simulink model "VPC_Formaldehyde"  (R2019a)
settings: Solver=VariableStepAuto  StartTime=0.0  StopTime=tend  RelTol=1e-3
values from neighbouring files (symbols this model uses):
  c_MeOH_0 = m_MeOH_sp_0/(m_MeOH_sp_0+m_air_sp_0)    [Mixer_script.m]
  comp_actuator_0 = [z0actuator,comp_w0]    [Compressor_script.m]
  comp_actuator_par = [comp_act_Ga;comp_act_tau;comp_act_zeta]    [Compressor_script.m]
  comp_deltaP = 2.1    [Compressor_script.m]
  comp_p1 = [a0,a1,a2,a3,b0,b1,b2,c0,c1,c2]    [Compressor_script.m]
  comp_p2 = [rho_a, kappa_a, cp_a, R_a, T_amb, d_c]    [Compressor_script.m]
  I_0_compressor = 0.39275    [Compressor_script.m]
  I_0_valve = valve_z0/valve_act_Ga    (= 0.7)    [Valve_script.m]
  Kc_comp = tau_compfotd/(K_compfotd*(tauc_comp+theta_compfotd))    [Compressor_script.m]
  Kc_mtot_MeOH = tau_mtot_MeOH/(K_mtot_MeOH*(tauc_mtot_MeOH+theta_mtot_MeOH))    (= 0.0903815050899)    [Basic_outer_PID_script.m]
  Kc_rpm_MeOH_VPC = tau_rpm_MeOH_VPC/(K_rpm_MeOH_VPC*(tauc_rpm_MeOH_VPC+theta_rpm_MeOH_VPC))    (= 0.590361445783)    [Tuning_VPC_script.m]
  Kc_valve = tau_valvefotd/(K_valvefotd*(tauc_valve+theta_valvefotd))    [Valve_script.m]
  Kc_x_air = tau_x_air/(K_x_air*(tauc_x_air+theta_x_air))    (= -74361.4590706)    [Basic_outer_PID_script.m]
  KI_comp = Kc_comp/tauI_comp    [Compressor_script.m]
  KI_mtot_MeOH = Kc_mtot_MeOH/tauI_mtot_MeOH    [Basic_outer_PID_script.m]
  KI_rpm_MeOH_VPC = Kc_rpm_MeOH_VPC/tauI_rpm_MeOH_SRC    [Tuning_VPC_script.m]
  KI_valve = Kc_valve/tauI_valve    [Valve_script.m]
  KI_x_air = Kc_x_air/tauI_x_air    [Basic_outer_PID_script.m]
  m_air_sp_0 = 23920    [Compressor_script.m]
  m_MeOH_bias = (MW_MeOH/MW_air)*mair_max*(x_MeOHsp/(1-x_MeOHsp))    [Bias_calc.m]    (also in Tuning_VPC_script.m = 2844.3)
  m_MeOH_sp_0 = 2940    [Valve_script.m]
  m_MeOH_sp_step = -m_MeOH_sp_0*0.1    [main_VPC_formaldehyde.m]    (also in main_basic_formaldehyde.m; main_basicTPM_formaldehyde.m)
  m_MeOH_sp_step_time = 20    [main_VPC_formaldehyde.m]    (also in main_basic_formaldehyde.m; main_basicTPM_formaldehyde.m)
  m_tot_sp_0 = m_air_sp_0+m_MeOH_sp_0    [main_VPC_formaldehyde.m]    (also in main_basic_formaldehyde.m; main_basicTPM_formaldehyde.m)
  m_tot_sp_step1 = 0*m_tot_sp_0*0.15    [main_VPC_formaldehyde.m]    (also in main_basic_formaldehyde.m; main_basicTPM_formaldehyde.m)
  m_tot_sp_step2 = 1*m_tot_sp_0*0.10    [main_VPC_formaldehyde.m]    (also in main_basic_formaldehyde.m; main_basicTPM_formaldehyde.m)
  m_tot_sp_step3 = 0*(m_tot_sp_step2+m_tot_sp_step1)    [main_VPC_formaldehyde.m]    (also in main_basic_formaldehyde.m = -1*(m_tot_sp_step2+m_tot_sp_step1); main_basicTPM_formaldehyde.m = -1*(m_tot_sp_step2+m_tot_sp_step1))
  m_tot_sp_step_t1 = 20    [main_VPC_formaldehyde.m]    (also in main_basic_formaldehyde.m; main_basicTPM_formaldehyde.m)
  m_tot_sp_step_t2 = 30    [main_VPC_formaldehyde.m]    (also in main_basic_formaldehyde.m; main_basicTPM_formaldehyde.m)
  m_tot_sp_step_t3 = 60    [main_VPC_formaldehyde.m]    (also in main_basic_formaldehyde.m = 70; main_basicTPM_formaldehyde.m = 70)
  max_air_PI = mair_max-m_air_sp_0    [Basic_outer_PID_script.m]
  max_MeOH_PI = m_MeOH_max-m_MeOH_sp_0    [Basic_outer_PID_script.m]
  min_air_PI = mair_min-m_air_sp_0    [Basic_outer_PID_script.m]
  min_MeOH_PI = m_MeOH_min-m_MeOH_sp_0    [Basic_outer_PID_script.m]
  N_cmax = 10048    [Compressor_script.m]
  N_cmin = 7500    [Compressor_script.m]
  N_max_PI = N_cmax-Nc_0    [Tuning_VPC_script.m]
  N_min_PI = -(Nc_0-N_cmin)    [Tuning_VPC_script.m]
  p_mix = [MW_MeOH;MW_air;rho_MeOH;rho_a;V_mixer]    [Mixer_script.m]
  PI_comp_max = 0.2    [Compressor_script.m]
  PI_comp_min = -I_0_compressor    (= -0.39275)    [Compressor_script.m]
  rpm_comp_sp = 0.95*N_cmax    [Tuning_VPC_script.m]
  valve_actuator_0 = [valve_z0 valve_w0]    [Valve_script.m]
  valve_actuator_par = [valve_act_Ga;valve_act_tau;valve_act_zeta]    [Valve_script.m]
  valve_Cv = m_MeOH_max/sqrt(valve_delta_p)    [Valve_script.m]
  valve_delta_p = 0.5    [Valve_script.m]
  valve_type = 3    [Valve_script.m]
  x_MeOH_sp_step1 = 1*-0.005    (= -0.005)    [main_VPC_formaldehyde.m]    (also in main_basic_formaldehyde.m; main_basicTPM_formaldehyde.m)
  x_MeOH_sp_step2 = 0*-0.005    (= 0)    [main_VPC_formaldehyde.m]    (also in main_basic_formaldehyde.m; main_basicTPM_formaldehyde.m)
  x_MeOH_sp_step3 = 0*+0.01    (= 0)    [main_VPC_formaldehyde.m]    (also in main_basic_formaldehyde.m; main_basicTPM_formaldehyde.m)
  x_MeOH_sp_step_t1 = 10    [main_VPC_formaldehyde.m]    (also in main_basic_formaldehyde.m; main_basicTPM_formaldehyde.m)
  x_MeOH_sp_step_t2 = 40    [main_VPC_formaldehyde.m]    (also in main_basic_formaldehyde.m; main_basicTPM_formaldehyde.m)
  x_MeOH_sp_step_t3 = 60    [main_VPC_formaldehyde.m]    (also in main_basic_formaldehyde.m = 70; main_basicTPM_formaldehyde.m = 70)
  x_MeOHsp_0 = 0.1    [main_VPC_formaldehyde.m]    (also in main_basic_formaldehyde.m; main_basicTPM_formaldehyde.m)
undefined symbols (not defined in the file or in its folder): actuator, compressor, mixerMeOH_O2_dynamic, mixerMeOH_O2_ss, valve
libraries: simulink x5

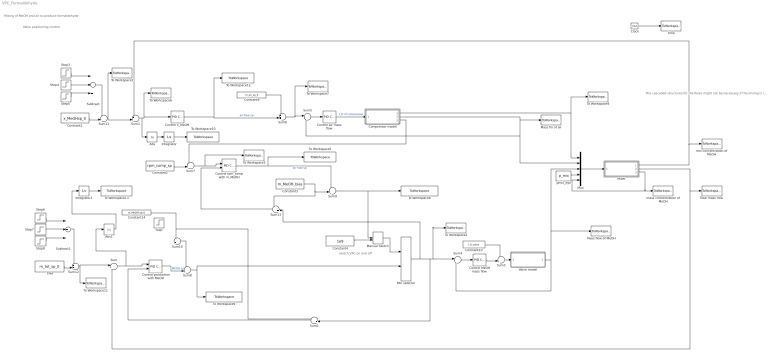
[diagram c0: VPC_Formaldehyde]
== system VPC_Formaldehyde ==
  note: Mixing of MeOH and air to produce formaldehyde
  note: The cascaded structures for the flows might not be necessary if the mixing is instantaneous. I just added them to have a general structure. I also added a small residence time in the tank.
  note: switch VPC on and off
  note: Valve positioning control
  Abs : Abs
  Abs1 : Abs
  Clock : Clock
  Compressor model : Subsystem
  Constant1 : Constant  Value=x_MeOHsp_0
  Constant10 : Constant  Value=I_0_valve
  Constant14 : Constant  Value=m_MeOH_sp_0
  Constant2 : Constant  Value=rpm_comp_sp
  Constant3 : Constant  Value=m_MeOH_bias
  Constant4 : Constant  Value=1e9
  Constant6 : Constant  Value=m_air_sp_0
  Control MeOH mass flow : simulink/Continuous/PID Controller  Controller=PI  Form=Parallel  TimeDomain=Continuous-time  SampleTime=-1  IntegratorMethod=Forward Euler  FilterMethod=Forward Euler  ControllerParametersSource=internal  P=Kc_valve  I=KI_valve  D=0  UseFilter=on  N=100  TunerSelectOption=Transfer Function Based (PID Tuner App)  InitialConditionSource=internal  InitialConditionForIntegrator=0  InitialConditionForFilter=0  DifferentiatorICPrevScaledInput=0  ExternalReset=none  TrackingMode=off  Kt=1  LimitOutput=on  UpperSaturationLimit=1-I_0_valve  LowerSaturationLimit=-I_0_valve  LinearizeAsGain=on  AntiWindupMode=back-calculation  Kb=1  POutMin=[]  POutMax=[]  IOutMin=[]  IOutMax=[]  DOutMin=[]  DOutMax=[]  NOutMin=[]  NOutMax=[]  SumOutMin=[]  SumOutMax=[]  SaturationOutMin=[]  SaturationOutMax=[]  PParamMin=[]  PParamMax=[]  IParamMin=[]  IParamMax=[]  DParamMin=[]  DParamMax=[]  NParamMin=[]  NParamMax=[]  KbParamMin=[]  KbParamMax=[]  KtParamMin=[]  KtParamMax=[]  KbOutMin=[]  KbOutMax=[]  KtOutMin=[]  KtOutMax=[]  IntegratorOutMin=[]  IntegratorOutMax=[]  FilterOutMin=[]  FilterOutMax=[]  SumI1OutMin=[]  SumI1OutMax=[]  SumI2OutMin=[]  SumI2OutMax=[]  SumI3OutMin=[]  SumI3OutMax=[]  SumI4OutMin=[]  SumI4OutMax=[]  SumDOutMin=[]  SumDOutMax=[]  DifferentiatorOutMin=[]  DifferentiatorOutMax=[]  FilterDiffOutCoefMin=[]  FilterDiffOutCoefMax=[]  ReciprocalOutMin=[]  ReciprocalOutMax=[]  SumDenOutMin=[]  SumDenOutMax=[]  SumNumOutMin=[]  SumNumOutMax=[]  DivideOutMin=[]  DivideOutMax=[]  IntegratorContinuousStateAttributes=''  IntegratorStateMustResolveToSignalObject=off  IntegratorRTWStateStorageClass=Auto  FilterContinuousStateAttributes=''  FilterStateMustResolveToSignalObject=off  FilterRTWStateStorageClass=Auto  ParallelPVariant=InternalParameters  IdealPVariant=Disabled  IVariant=InternalParameters  DVariant=Disabled  IntegratorVariant=Continuous  SatVariant=Enabled  AWVariant=BackCalculation  PCopyVariant=Disabled  TRVariant=Disabled  FdbkBlocksVariant=Forward  IdealPFdbkVariant=Disabled  SatFdbkVariant=Disabled  DerivativeFilterVariant=Disabled  NVariant=Disabled  NCopyVariant=Disabled_SignalSpec  FilterICVariant=Disabled  IntegratorICVariant=InternalICs  ExternalResetVariant=Disabled  TRSumVariant=Passthrough  SumFdbkVariant=Disabled  SumVariant=Sum_PI
  Control air mass flow : simulink/Continuous/PID Controller  Controller=PI  Form=Parallel  TimeDomain=Continuous-time  SampleTime=-1  IntegratorMethod=Forward Euler  FilterMethod=Forward Euler  ControllerParametersSource=internal  P=Kc_comp  I=KI_comp  D=0  UseFilter=on  N=100  TunerSelectOption=Transfer Function Based (PID Tuner App)  InitialConditionSource=internal  InitialConditionForIntegrator=0  InitialConditionForFilter=0  DifferentiatorICPrevScaledInput=0  ExternalReset=none  TrackingMode=off  Kt=1  LimitOutput=on  UpperSaturationLimit=PI_comp_max  LowerSaturationLimit=PI_comp_min  LinearizeAsGain=on  AntiWindupMode=back-calculation  Kb=1  POutMin=[]  POutMax=[]  IOutMin=[]  IOutMax=[]  DOutMin=[]  DOutMax=[]  NOutMin=[]  NOutMax=[]  SumOutMin=[]  SumOutMax=[]  SaturationOutMin=[]  SaturationOutMax=[]  PParamMin=[]  PParamMax=[]  IParamMin=[]  IParamMax=[]  DParamMin=[]  DParamMax=[]  NParamMin=[]  NParamMax=[]  KbParamMin=[]  KbParamMax=[]  KtParamMin=[]  KtParamMax=[]  KbOutMin=[]  KbOutMax=[]  KtOutMin=[]  KtOutMax=[]  IntegratorOutMin=[]  IntegratorOutMax=[]  FilterOutMin=[]  FilterOutMax=[]  SumI1OutMin=[]  SumI1OutMax=[]  SumI2OutMin=[]  SumI2OutMax=[]  SumI3OutMin=[]  SumI3OutMax=[]  SumI4OutMin=[]  SumI4OutMax=[]  SumDOutMin=[]  SumDOutMax=[]  DifferentiatorOutMin=[]  DifferentiatorOutMax=[]  FilterDiffOutCoefMin=[]  FilterDiffOutCoefMax=[]  ReciprocalOutMin=[]  ReciprocalOutMax=[]  SumDenOutMin=[]  SumDenOutMax=[]  SumNumOutMin=[]  SumNumOutMax=[]  DivideOutMin=[]  DivideOutMax=[]  IntegratorContinuousStateAttributes=''  IntegratorStateMustResolveToSignalObject=off  IntegratorRTWStateStorageClass=Auto  FilterContinuousStateAttributes=''  FilterStateMustResolveToSignalObject=off  FilterRTWStateStorageClass=Auto  ParallelPVariant=InternalParameters  IdealPVariant=Disabled  IVariant=InternalParameters  DVariant=Disabled  IntegratorVariant=Continuous  SatVariant=Enabled  AWVariant=BackCalculation  PCopyVariant=Disabled  TRVariant=Disabled  FdbkBlocksVariant=Forward  IdealPFdbkVariant=Disabled  SatFdbkVariant=Disabled  DerivativeFilterVariant=Disabled  NVariant=Disabled  NCopyVariant=Disabled_SignalSpec  FilterICVariant=Disabled  IntegratorICVariant=InternalICs  ExternalResetVariant=Disabled  TRSumVariant=Passthrough  SumFdbkVariant=Disabled  SumVariant=Sum_PI
  Control production with MeOH : simulink/Continuous/PID Controller  Controller=PI  Form=Parallel  TimeDomain=Continuous-time  SampleTime=-1  IntegratorMethod=Forward Euler  FilterMethod=Forward Euler  ControllerParametersSource=internal  P=Kc_mtot_MeOH  I=KI_mtot_MeOH  D=0  UseFilter=on  N=100  TunerSelectOption=Transfer Function Based (PID Tuner App)  InitialConditionSource=internal  InitialConditionForIntegrator=0  InitialConditionForFilter=0  DifferentiatorICPrevScaledInput=0  ExternalReset=none  TrackingMode=on  Kt=1  LimitOutput=on  UpperSaturationLimit=max_MeOH_PI  LowerSaturationLimit=min_MeOH_PI  LinearizeAsGain=on  AntiWindupMode=back-calculation  Kb=1  POutMin=[]  POutMax=[]  IOutMin=[]  IOutMax=[]  DOutMin=[]  DOutMax=[]  NOutMin=[]  NOutMax=[]  SumOutMin=[]  SumOutMax=[]  SaturationOutMin=[]  SaturationOutMax=[]  PParamMin=[]  PParamMax=[]  IParamMin=[]  IParamMax=[]  DParamMin=[]  DParamMax=[]  NParamMin=[]  NParamMax=[]  KbParamMin=[]  KbParamMax=[]  KtParamMin=[]  KtParamMax=[]  KbOutMin=[]  KbOutMax=[]  KtOutMin=[]  KtOutMax=[]  IntegratorOutMin=[]  IntegratorOutMax=[]  FilterOutMin=[]  FilterOutMax=[]  SumI1OutMin=[]  SumI1OutMax=[]  SumI2OutMin=[]  SumI2OutMax=[]  SumI3OutMin=[]  SumI3OutMax=[]  SumI4OutMin=[]  SumI4OutMax=[]  SumDOutMin=[]  SumDOutMax=[]  DifferentiatorOutMin=[]  DifferentiatorOutMax=[]  FilterDiffOutCoefMin=[]  FilterDiffOutCoefMax=[]  ReciprocalOutMin=[]  ReciprocalOutMax=[]  SumDenOutMin=[]  SumDenOutMax=[]  SumNumOutMin=[]  SumNumOutMax=[]  DivideOutMin=[]  DivideOutMax=[]  IntegratorContinuousStateAttributes=''  IntegratorStateMustResolveToSignalObject=off  IntegratorRTWStateStorageClass=Auto  FilterContinuousStateAttributes=''  FilterStateMustResolveToSignalObject=off  FilterRTWStateStorageClass=Auto  ParallelPVariant=InternalParameters  IdealPVariant=Disabled  IVariant=InternalParameters  DVariant=Disabled  IntegratorVariant=Continuous  SatVariant=Enabled  AWVariant=BackCalculation  PCopyVariant=Disabled  TRVariant=Enabled  FdbkBlocksVariant=Forward  IdealPFdbkVariant=Disabled  SatFdbkVariant=Disabled  DerivativeFilterVariant=Disabled  NVariant=Disabled  NCopyVariant=Disabled_SignalSpec  FilterICVariant=Disabled  IntegratorICVariant=InternalICs  ExternalResetVariant=Disabled  TRSumVariant=TrackingMode  SumFdbkVariant=Disabled  SumVariant=Sum_PI
  Control rpm_comp with m_MeOH : simulink/Continuous/PID Controller  Controller=PI  Form=Parallel  TimeDomain=Continuous-time  SampleTime=-1  IntegratorMethod=Forward Euler  FilterMethod=Forward Euler  ControllerParametersSource=internal  P=Kc_rpm_MeOH_VPC  I=KI_rpm_MeOH_VPC  D=0  UseFilter=on  N=100  TunerSelectOption=Transfer Function Based (PID Tuner App)  InitialConditionSource=internal  InitialConditionForIntegrator=0  InitialConditionForFilter=0  DifferentiatorICPrevScaledInput=0  ExternalReset=none  TrackingMode=on  Kt=1  LimitOutput=on  UpperSaturationLimit=N_max_PI  LowerSaturationLimit=N_min_PI  LinearizeAsGain=on  AntiWindupMode=back-calculation  Kb=1  POutMin=[]  POutMax=[]  IOutMin=[]  IOutMax=[]  DOutMin=[]  DOutMax=[]  NOutMin=[]  NOutMax=[]  SumOutMin=[]  SumOutMax=[]  SaturationOutMin=[]  SaturationOutMax=[]  PParamMin=[]  PParamMax=[]  IParamMin=[]  IParamMax=[]  DParamMin=[]  DParamMax=[]  NParamMin=[]  NParamMax=[]  KbParamMin=[]  KbParamMax=[]  KtParamMin=[]  KtParamMax=[]  KbOutMin=[]  KbOutMax=[]  KtOutMin=[]  KtOutMax=[]  IntegratorOutMin=[]  IntegratorOutMax=[]  FilterOutMin=[]  FilterOutMax=[]  SumI1OutMin=[]  SumI1OutMax=[]  SumI2OutMin=[]  SumI2OutMax=[]  SumI3OutMin=[]  SumI3OutMax=[]  SumI4OutMin=[]  SumI4OutMax=[]  SumDOutMin=[]  SumDOutMax=[]  DifferentiatorOutMin=[]  DifferentiatorOutMax=[]  FilterDiffOutCoefMin=[]  FilterDiffOutCoefMax=[]  ReciprocalOutMin=[]  ReciprocalOutMax=[]  SumDenOutMin=[]  SumDenOutMax=[]  SumNumOutMin=[]  SumNumOutMax=[]  DivideOutMin=[]  DivideOutMax=[]  IntegratorContinuousStateAttributes=''  IntegratorStateMustResolveToSignalObject=off  IntegratorRTWStateStorageClass=Auto  FilterContinuousStateAttributes=''  FilterStateMustResolveToSignalObject=off  FilterRTWStateStorageClass=Auto  ParallelPVariant=InternalParameters  IdealPVariant=Disabled  IVariant=InternalParameters  DVariant=Disabled  IntegratorVariant=Continuous  SatVariant=Enabled  AWVariant=BackCalculation  PCopyVariant=Disabled  TRVariant=Enabled  FdbkBlocksVariant=Forward  IdealPFdbkVariant=Disabled  SatFdbkVariant=Disabled  DerivativeFilterVariant=Disabled  NVariant=Disabled  NCopyVariant=Disabled_SignalSpec  FilterICVariant=Disabled  IntegratorICVariant=InternalICs  ExternalResetVariant=Disabled  TRSumVariant=TrackingMode  SumFdbkVariant=Disabled  SumVariant=Sum_PI
  "Control x_MeOH " : simulink/Continuous/PID Controller  Controller=PI  Form=Parallel  TimeDomain=Continuous-time  SampleTime=-1  IntegratorMethod=Forward Euler  FilterMethod=Forward Euler  ControllerParametersSource=internal  P=Kc_x_air  I=KI_x_air  D=0  UseFilter=on  N=100  TunerSelectOption=Transfer Function Based (PID Tuner App)  InitialConditionSource=internal  InitialConditionForIntegrator=0  InitialConditionForFilter=0  DifferentiatorICPrevScaledInput=0  ExternalReset=none  TrackingMode=off  Kt=1  LimitOutput=on  UpperSaturationLimit=max_air_PI  LowerSaturationLimit=min_air_PI  LinearizeAsGain=on  AntiWindupMode=back-calculation  Kb=1  POutMin=[]  POutMax=[]  IOutMin=[]  IOutMax=[]  DOutMin=[]  DOutMax=[]  NOutMin=[]  NOutMax=[]  SumOutMin=[]  SumOutMax=[]  SaturationOutMin=[]  SaturationOutMax=[]  PParamMin=[]  PParamMax=[]  IParamMin=[]  IParamMax=[]  DParamMin=[]  DParamMax=[]  NParamMin=[]  NParamMax=[]  KbParamMin=[]  KbParamMax=[]  KtParamMin=[]  KtParamMax=[]  KbOutMin=[]  KbOutMax=[]  KtOutMin=[]  KtOutMax=[]  IntegratorOutMin=[]  IntegratorOutMax=[]  FilterOutMin=[]  FilterOutMax=[]  SumI1OutMin=[]  SumI1OutMax=[]  SumI2OutMin=[]  SumI2OutMax=[]  SumI3OutMin=[]  SumI3OutMax=[]  SumI4OutMin=[]  SumI4OutMax=[]  SumDOutMin=[]  SumDOutMax=[]  DifferentiatorOutMin=[]  DifferentiatorOutMax=[]  FilterDiffOutCoefMin=[]  FilterDiffOutCoefMax=[]  ReciprocalOutMin=[]  ReciprocalOutMax=[]  SumDenOutMin=[]  SumDenOutMax=[]  SumNumOutMin=[]  SumNumOutMax=[]  DivideOutMin=[]  DivideOutMax=[]  IntegratorContinuousStateAttributes=''  IntegratorStateMustResolveToSignalObject=off  IntegratorRTWStateStorageClass=Auto  FilterContinuousStateAttributes=''  FilterStateMustResolveToSignalObject=off  FilterRTWStateStorageClass=Auto  ParallelPVariant=InternalParameters  IdealPVariant=Disabled  IVariant=InternalParameters  DVariant=Disabled  IntegratorVariant=Continuous  SatVariant=Enabled  AWVariant=BackCalculation  PCopyVariant=Disabled  TRVariant=Disabled  FdbkBlocksVariant=Forward  IdealPFdbkVariant=Disabled  SatFdbkVariant=Disabled  DerivativeFilterVariant=Disabled  NVariant=Disabled  NCopyVariant=Disabled_SignalSpec  FilterICVariant=Disabled  IntegratorICVariant=InternalICs  ExternalResetVariant=Disabled  TRSumVariant=Passthrough  SumFdbkVariant=Disabled  SumVariant=Sum_PI
  Integrator : Integrator
  Integrator1 : Integrator
  Manual Switch : ManualSwitch
  Mass flo of air : ToWorkspace  VariableName=m_air  SampleTime=-1
  Mass flow of MeOH : ToWorkspace  VariableName=m_MeOH  SampleTime=-1
  Min selector : MinMax  Inputs=2
  Mixer : Subsystem
  Mux : Mux  Inputs=5
  Step : Step  Time=m_MeOH_sp_step_time  After=m_MeOH_sp_step  SampleTime=0
  Step3 : Step  Time=x_MeOH_sp_step_t1  After=x_MeOH_sp_step1  SampleTime=0
  Step4 : Step  Time=x_MeOH_sp_step_t2  After=x_MeOH_sp_step2  SampleTime=0
  Step5 : Step  Time=x_MeOH_sp_step_t3  After=x_MeOH_sp_step3  SampleTime=0
  Step6 : Step  Time=m_tot_sp_step_t1  After=m_tot_sp_step1  SampleTime=0
  Step7 : Step  Time=m_tot_sp_step_t2  After=m_tot_sp_step2  SampleTime=0
  Step8 : Step  Time=m_tot_sp_step_t3  After=m_tot_sp_step3  SampleTime=0
  Subtract : Sum  Inputs=+++
  Subtract1 : Sum  Inputs=+++
  Sum : Sum  Inputs=|+-
  Sum{1..2,7,13} (4 alike) : Sum  Inputs=-+|
  Sum{3,6,8..12} (7 alike) : Sum  Inputs=++|
  Sum4 : Sum  Inputs=|+-
  Sum5 : Sum  Inputs=|+-
  TPM : Constant  Value=m_tot_sp_0
  To Workspace1 : ToWorkspace  VariableName=x_MeOHsp  SampleTime=-1
  To Workspace10 : ToWorkspace  VariableName=IAExMeOH  SampleTime=-1
  To Workspace11 : ToWorkspace  VariableName=m_tot_sp  SampleTime=-1
  To Workspace12 : ToWorkspace  VariableName=u_air  SampleTime=-1
  To Workspace13 : ToWorkspace  VariableName=IAEmtot  SampleTime=-1
  To Workspace2 : ToWorkspace  VariableName=m_MEOH_sp  SampleTime=-1
  To Workspace3 : ToWorkspace  VariableName=rpm_error  SampleTime=-1
  To Workspace4 : ToWorkspace  VariableName=Q_air  SampleTime=-1
  To Workspace5 : ToWorkspace  VariableName=u_MeOH  SampleTime=-1
  To Workspace6 : ToWorkspace  VariableName=x_MeOH_error  SampleTime=-1
  To Workspace7 : ToWorkspace  VariableName=m_air_sp  SampleTime=-1
  To Workspace8 : ToWorkspace  VariableName=m_MEOH_sp_VPC  SampleTime=-1
  To Workspace9 : ToWorkspace  VariableName=m_MeOH_sp_m_tot  SampleTime=-1
  Total mass flow : ToWorkspace  VariableName=m_tot  SampleTime=-1
  Valve model : Subsystem
  mass concentration of MeOH : ToWorkspace  VariableName=c_MeOH  SampleTime=-1
  mol concentration of MeOH : ToWorkspace  VariableName=x_MeOH  SampleTime=-1
  pmix_dyn : Constant  Value=p_mix
  time : ToWorkspace  VariableName=t  SampleTime=-1
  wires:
  Valve model/1(m_MeOH) -> Mass flow of MeOH/1, Mux/3, Sum4/2
  Clock/1 -> time/1
  Compressor model/2(m_air) -> Sum5/2, Mux/2, Mass flo of air/1
  Compressor model/1(Q_air) -> Mux/1, To Workspace4/1
  Control MeOH mass flow/1 -> Sum3/2
  Constant10/1 -> Sum3/1
  Sum4/1 -> Control MeOH mass flow/1
  Mixer/2(m_tot) -> Total mass flow/1, Sum/2
  Mixer/1(x_MeOH) -> Sum1/1, mol concentration of MeOH/1
  pmix_dyn/1 -> Mux/4
  Constant1/1 -> Sum11/2
  Step3/1 -> Subtract/1
  Step4/1 -> Subtract/2
  Step5/1 -> Subtract/3
  TPM/1 -> Sum12/2
  Sum12/1 -> To Workspace11/1, Sum/1
  Step6/1 -> Subtract1/1
  Step7/1 -> Subtract1/2
  Step8/1 -> Subtract1/3
  Subtract1/1 -> Sum12/1
  Control air mass flow/1 -> Compressor model/1(I_blower)  "I_O of compressor"
  Sum5/1 -> Control air mass flow/1
  Mux/1 -> Mixer/1(Mix_par)
  Mixer/3(c_MeOH) -> Mux/5, mass concentration of MeOH/1
  Sum3/1 -> Valve model/1(I_valve)
  Sum8/1 -> To Workspace9/1, Min selector/2
  Min selector/1 -> Sum13/2, Sum2/2, To Workspace2/1, Sum4/1
  Subtract/1 -> Sum11/1
  Constant14/1 -> Sum2/1, Sum10/1
  Sum2/1 -> Control production with MeOH/2
  Sum1/1 -> Abs/1, To Workspace6/1, "Control x_MeOH "/1
  Sum6/1 -> Sum5/1, To Workspace7/1
  "Control x_MeOH "/1 -> To Workspace12/1, Sum6/2  "air flow sp"
  Constant6/1 -> Sum6/1
  Constant2/1 -> Sum7/2
  Compressor model/3(rpm_comp) -> Sum7/1
  Sum7/1 -> To Workspace3/1, Control rpm_comp with m_MeOH/1
  Control rpm_comp with m_MeOH/1 -> Sum9/1, To Workspace5/1  "air flow sp"
  Constant3/1 -> Sum9/2, Sum13/1
  Sum9/1 -> Manual Switch/1, To Workspace8/1
  Manual Switch/1 -> Min selector/1
  Constant4/1 -> Manual Switch/2
  Sum11/1 -> To Workspace1/1, Sum1/2
  Sum10/1 -> Sum8/1
  Sum13/1 -> Control rpm_comp with m_MeOH/2
  Control production with MeOH/1 -> Sum8/2  "MEOH sp"
  Abs/1 -> Integrator/1
  Abs1/1 -> Integrator1/1
  Sum/1 -> Abs1/1, Control production with MeOH/1
  Integrator/1 -> To Workspace10/1
  Integrator1/1 -> To Workspace13/1

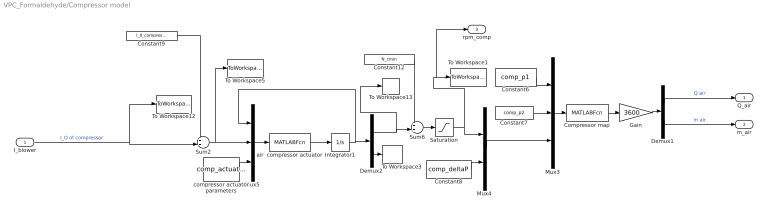
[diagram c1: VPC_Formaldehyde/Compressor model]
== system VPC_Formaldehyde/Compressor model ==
  I_blower : Inport
  Compressor map : MATLABFcn  MATLABFcn=compressor(u(1:10),u(11:16),u(17:18))  OutputDimensions=2
  Constant12 : Constant  Value=N_cmin
  Constant6 : Constant  Value=comp_p1
  Constant7 : Constant  Value=comp_p2
  Constant8 : Constant  Value=comp_deltaP
  Constant9 : Constant  Value=I_0_compressor
  Demux1 : Demux  Outputs=2
  Demux2 : Demux  Outputs=2
  Gain : Gain  Gain=3600
  Integrator1 : Integrator  InitialCondition=comp_actuator_0
  Mux3 : Mux  Inputs=3
  Mux4 : Mux  Inputs=2
  Mux5 : Mux  Inputs=3
  Saturation : Saturate  UpperLimit=N_cmax  LowerLimit=N_cmin
  Sum2 : Sum  Inputs=++|
  Sum6 : Sum  Inputs=++|
  To Workspace1 : ToWorkspace  VariableName=comp_rpm  SampleTime=-1
  To Workspace12 : ToWorkspace  VariableName=I_air0  SampleTime=-1
  To Workspace13 : ToWorkspace  VariableName=Nc_act1  SampleTime=-1
  To Workspace3 : ToWorkspace  VariableName=wcomp  SampleTime=-1
  To Workspace5 : ToWorkspace  VariableName=I_air  SampleTime=-1
  air  compressor actuator : MATLABFcn  MATLABFcn=actuator(u(1:2),u(3),u(4:6))  OutputDimensions=2
  compressor actuator parameters : Constant  Value=comp_actuator_par
  Q_air : Outport
  m_air : Outport  Port=2
  rpm_comp : Outport  Port=3
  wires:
  I_blower/1 -> To Workspace12/1, Sum2/2  "I_O of compressor"
  Constant9/1 -> Sum2/1
  Sum6/1 -> Saturation/1
  Constant12/1 -> Sum6/1
  Constant6/1 -> Mux3/1
  Mux5/1 -> air  compressor actuator/1
  Sum2/1 -> To Workspace5/1, Mux5/2
  Integrator1/1 -> Demux2/1, Mux5/1
  Demux2/1 -> To Workspace13/1, Sum6/2
  air  compressor actuator/1 -> Integrator1/1
  Constant8/1 -> Mux4/2
  Demux2/2 -> To Workspace3/1
  Demux1/1 -> Q_air/1  "Q air"
  Mux3/1 -> Compressor map/1
  Constant7/1 -> Mux3/2
  Mux4/1 -> Mux3/3
  Saturation/1 -> rpm_comp/1, To Workspace1/1, Mux4/1
  Compressor map/1 -> Gain/1
  Gain/1 -> Demux1/1
  Demux1/2 -> m_air/1  "m air"
  compressor actuator parameters/1 -> Mux5/3

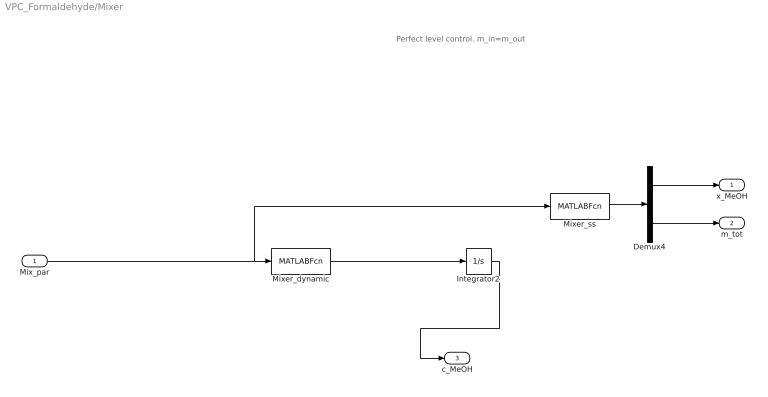
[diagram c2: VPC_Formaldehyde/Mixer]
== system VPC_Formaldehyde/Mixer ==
  note: Perfect level control. m_in=m_out
  Mix_par : Inport
  Demux4 : Demux  Outputs=2
  Integrator2 : Integrator  InitialCondition=c_MeOH_0
  Mixer_dynamic : MATLABFcn  MATLABFcn=mixerMeOH_O2_dynamic(u(1:3),u(4:8),u(9))  OutputDimensions=1
  Mixer_ss : MATLABFcn  MATLABFcn=mixerMeOH_O2_ss(u(1:3),u(4:8),u(9))  OutputDimensions=2
  x_MeOH : Outport
  m_tot : Outport  Port=2
  c_MeOH : Outport  Port=3
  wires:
  Integrator2/1 -> c_MeOH/1
  Mix_par/1 -> Mixer_ss/1, Mixer_dynamic/1
  Mixer_dynamic/1 -> Integrator2/1
  Mixer_ss/1 -> Demux4/1
  Demux4/1 -> x_MeOH/1
  Demux4/2 -> m_tot/1

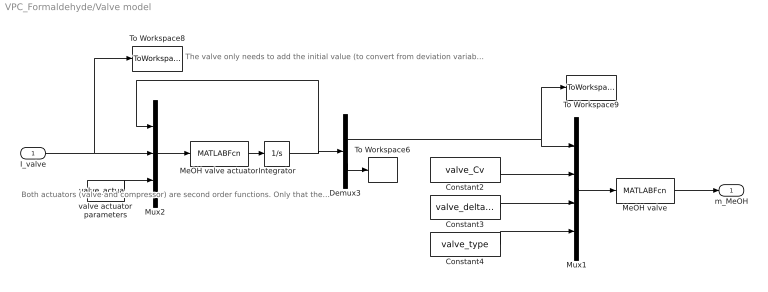
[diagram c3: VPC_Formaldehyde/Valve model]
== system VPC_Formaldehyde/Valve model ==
  note: The valve only needs to add the initial value (to convert from deviation variables to actual variables "once" before the actuator. The compressor also needs it before the actuator because the range does not start in 0. (Maybe there is a better way to do this).
  note: Both actuators (valve and compressor) are second order functions. Only that the time constants and the damping factors are different.
  I_valve : Inport
  Constant2 : Constant  Value=valve_Cv
  Constant3 : Constant  Value=valve_delta_p
  Constant4 : Constant  Value=valve_type
  Demux3 : Demux  Outputs=2
  Integrator : Integrator  InitialCondition=valve_actuator_0
  MeOH valve : MATLABFcn  MATLABFcn=valve(u)  OutputDimensions=1
  MeOH valve actuator : MATLABFcn  MATLABFcn=actuator(u(1:2),u(3),u(4:6))  OutputDimensions=2
  Mux1 : Mux
  Mux2 : Mux  Inputs=3
  To Workspace6 : ToWorkspace  VariableName=wvalve  SampleTime=-1
  To Workspace8 : ToWorkspace  VariableName=I_MeOH  SampleTime=-1
  To Workspace9 : ToWorkspace  VariableName=z_MeOH  SampleTime=-1
  valve actuator parameters : Constant  Value=valve_actuator_par
  m_MeOH : Outport
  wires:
  Demux3/2 -> To Workspace6/1
  Demux3/1 -> To Workspace9/1, Mux1/1
  MeOH valve actuator/1 -> Integrator/1
  Integrator/1 -> Demux3/1, Mux2/1
  Constant4/1 -> Mux1/4
  Constant3/1 -> Mux1/3
  I_valve/1 -> To Workspace8/1, Mux2/2
  Constant2/1 -> Mux1/2
  Mux2/1 -> MeOH valve actuator/1
  Mux1/1 -> MeOH valve/1
  valve actuator parameters/1 -> Mux2/3
  MeOH valve/1 -> m_MeOH/1
